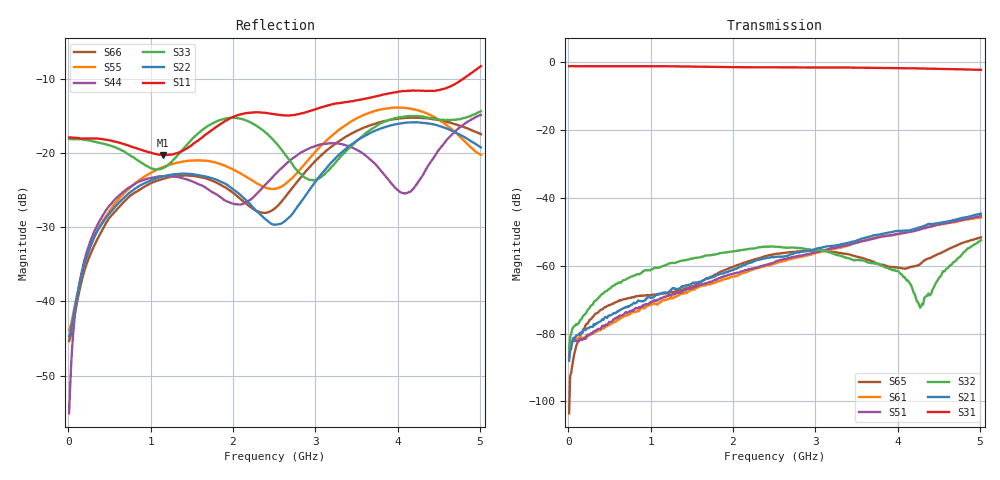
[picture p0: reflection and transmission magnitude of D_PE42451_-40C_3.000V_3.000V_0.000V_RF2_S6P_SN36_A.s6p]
! Device ID: PE42451
! Serial: 36
! Insertion: A
! Temp: -40C
! VDD: 3.000
! Control_Hi: 100.000
! Control_Lo: 0.000
! Logic State: RF2
! Port 1: RFC
! Port 2: RF1
! Port 3: RF2
! Port 4: RF3
! Port 5: RF4
! Port 6: RF5
! V1 = 0.00
! V2 = 3.00
! V3 = 0.00
! V4 = 0.00
! IDD: 1.323780e-05
#  Hz  S  RI  R  50
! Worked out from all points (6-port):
!   401 points, 10 MHz to 5.01 GHz, reference 50 ohm
!   strongest paths, dB at 10 MHz, 1.26 GHz, 2.51 GHz, 3.76 GHz, 5.01 GHz:
!     S31: -1.3, -1.3, -1.6, -1.8, -2.3
!     S21: -88.0, -66.8, -57.5, -50.9, -44.7
!     S32: -84.5, -59.2, -54.5, -59.4, -52.5
!     S51: -87.1, -68.5, -58.9, -51.8, -45.5
!     S61: -86.8, -69.7, -59.3, -51.5, -45.8
!     S65: -103.5, -67.8, -56.6, -59.6, -51.7
!   lowest |S11| = -20.3 dB at 1.147 GHz (marker M1), VSWR 1.21, Z = 56.9 - j7.76 ohm
!   |S11| at or under -10 dB: start of sweep to 4.797 GHz
